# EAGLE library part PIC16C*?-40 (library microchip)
MICROCONTROLLER 8-Bit CMOS Pin compatible: PIC16CR64, PIC16C64A, PIC16C65A, PIC16CR65, PIC16C67, PIC16C74A, PIC16C77
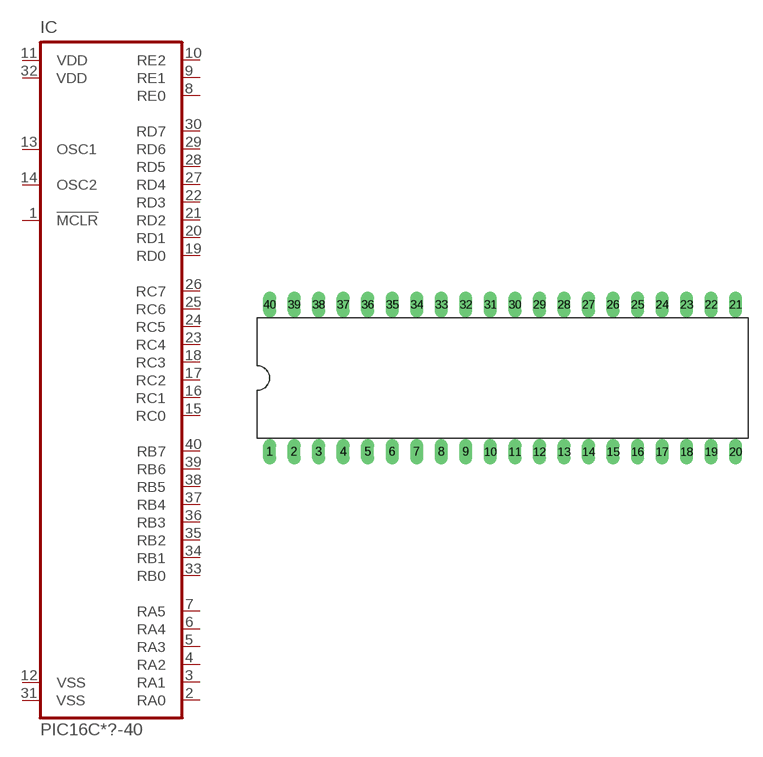
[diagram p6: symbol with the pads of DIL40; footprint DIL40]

Designator prefix IC

## PIC16C64AP-40 (MPN: PIC16C64A-04I/P; OC_FARNELL: 1084225; OC_NEWARK: 24M5871), PIC16C65AP-40 (MPN: PIC16C65A-04/P; OC_FARNELL: 9759670; OC_NEWARK: 97K7249), PIC16C67P-40 (MF: MICROCHIP; MPN: PIC16C67-20/P; OC_FARNELL: 9759751; OC_NEWARK: 72K7295), PIC16C74AP-40 (MPN: PIC16C74A-04I/P; OC_FARNELL: 9760059; OC_NEWARK: 31M5834), PIC16C77P-40 (MF: MICROCHIP; MPN: PIC16C77-20I/P; OC_FARNELL: 9760172; OC_NEWARK: 96K3855), PIC16CR64P-40 (OC_FARNELL: unknown; OC_NEWARK: unknown), PIC16CR65P-40 (OC_FARNELL: unknown; OC_NEWARK: unknown)  [DIL40]
1  !MCLR  in
2  RA0
3  RA1
4  RA2
5  RA3
6  RA4
7  RA5
8  RE0
9  RE1
10  RE2
11  VDD  pwr
12  VSS  pwr
13  OSC1  in
14  OSC2  out
15  RC0  out
16  RC1  out
17  RC2  out
18  RC3  out
19  RD0
20  RD1
21  RD2
22  RD3
23  RC4  out
24  RC5  out
25  RC6  out
26  RC7  out
27  RD4
28  RD5
29  RD6
30  RD7
31  VSS  pwr
32  VDD  pwr
33  RB0
34  RB1
35  RB2
36  RB3
37  RB4
38  RB5
39  RB6
40  RB7

## PIC16C64AJW-40 (MPN: PIC16C64A-04I/P; OC_FARNELL: 1084225; OC_NEWARK: 24M5871), PIC16C65AJW-40 (MPN: PIC16C65A-04/P; OC_FARNELL: 9759670; OC_NEWARK: 97K7249), PIC16C67JW-40 (MF: MICROCHIP; MPN: PIC16C67-04/P; OC_FARNELL: 9759751; OC_NEWARK: 61K3443), PIC16C74AJW-40 (MPN: PIC16C74A-10/P; OC_FARNELL: 1084347; OC_NEWARK: 97K7294), PIC16C77JW-40 (MF: MICROCHIP; MPN: PIC16C77-20/P; OC_FARNELL: 9760172; OC_NEWARK: 12C1937), PIC16CR64JW-40 (OC_FARNELL: unknown; OC_NEWARK: unknown), PIC16CR65JW-40 (OC_FARNELL: unknown; OC_NEWARK: unknown)  [DIL40]
Pads as for DIL40

## Footprint DIL40 (pad centres in mm)
Dual In Line package type P
drill 0.813 long: 1 -24.13,-7.62; 2 -21.59,-7.62; 3 -19.05,-7.62; 4 -16.51,-7.62; 5 -13.97,-7.62; 6 -11.43,-7.62; 7 -8.89,-7.62; 8 -6.35,-7.62; 9 -3.81,-7.62; 10 -1.27,-7.62; 11 1.27,-7.62; 12 3.81,-7.62; 13 6.35,-7.62; 14 8.89,-7.62; 15 11.43,-7.62; 16 13.97,-7.62; 17 16.51,-7.62; 18 19.05,-7.62; 19 21.59,-7.62; 20 24.13,-7.62; 21 24.13,7.62; 22 21.59,7.62; 23 19.05,7.62; 24 16.51,7.62; 25 13.97,7.62; 26 11.43,7.62; 27 8.89,7.62; 28 6.35,7.62; 29 3.81,7.62; 30 1.27,7.62; 31 -1.27,7.62; 32 -3.81,7.62; 33 -6.35,7.62; 34 -8.89,7.62; 35 -11.43,7.62; 36 -13.97,7.62; 37 -16.51,7.62; 38 -19.05,7.62; 39 -21.59,7.62; 40 -24.13,7.62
